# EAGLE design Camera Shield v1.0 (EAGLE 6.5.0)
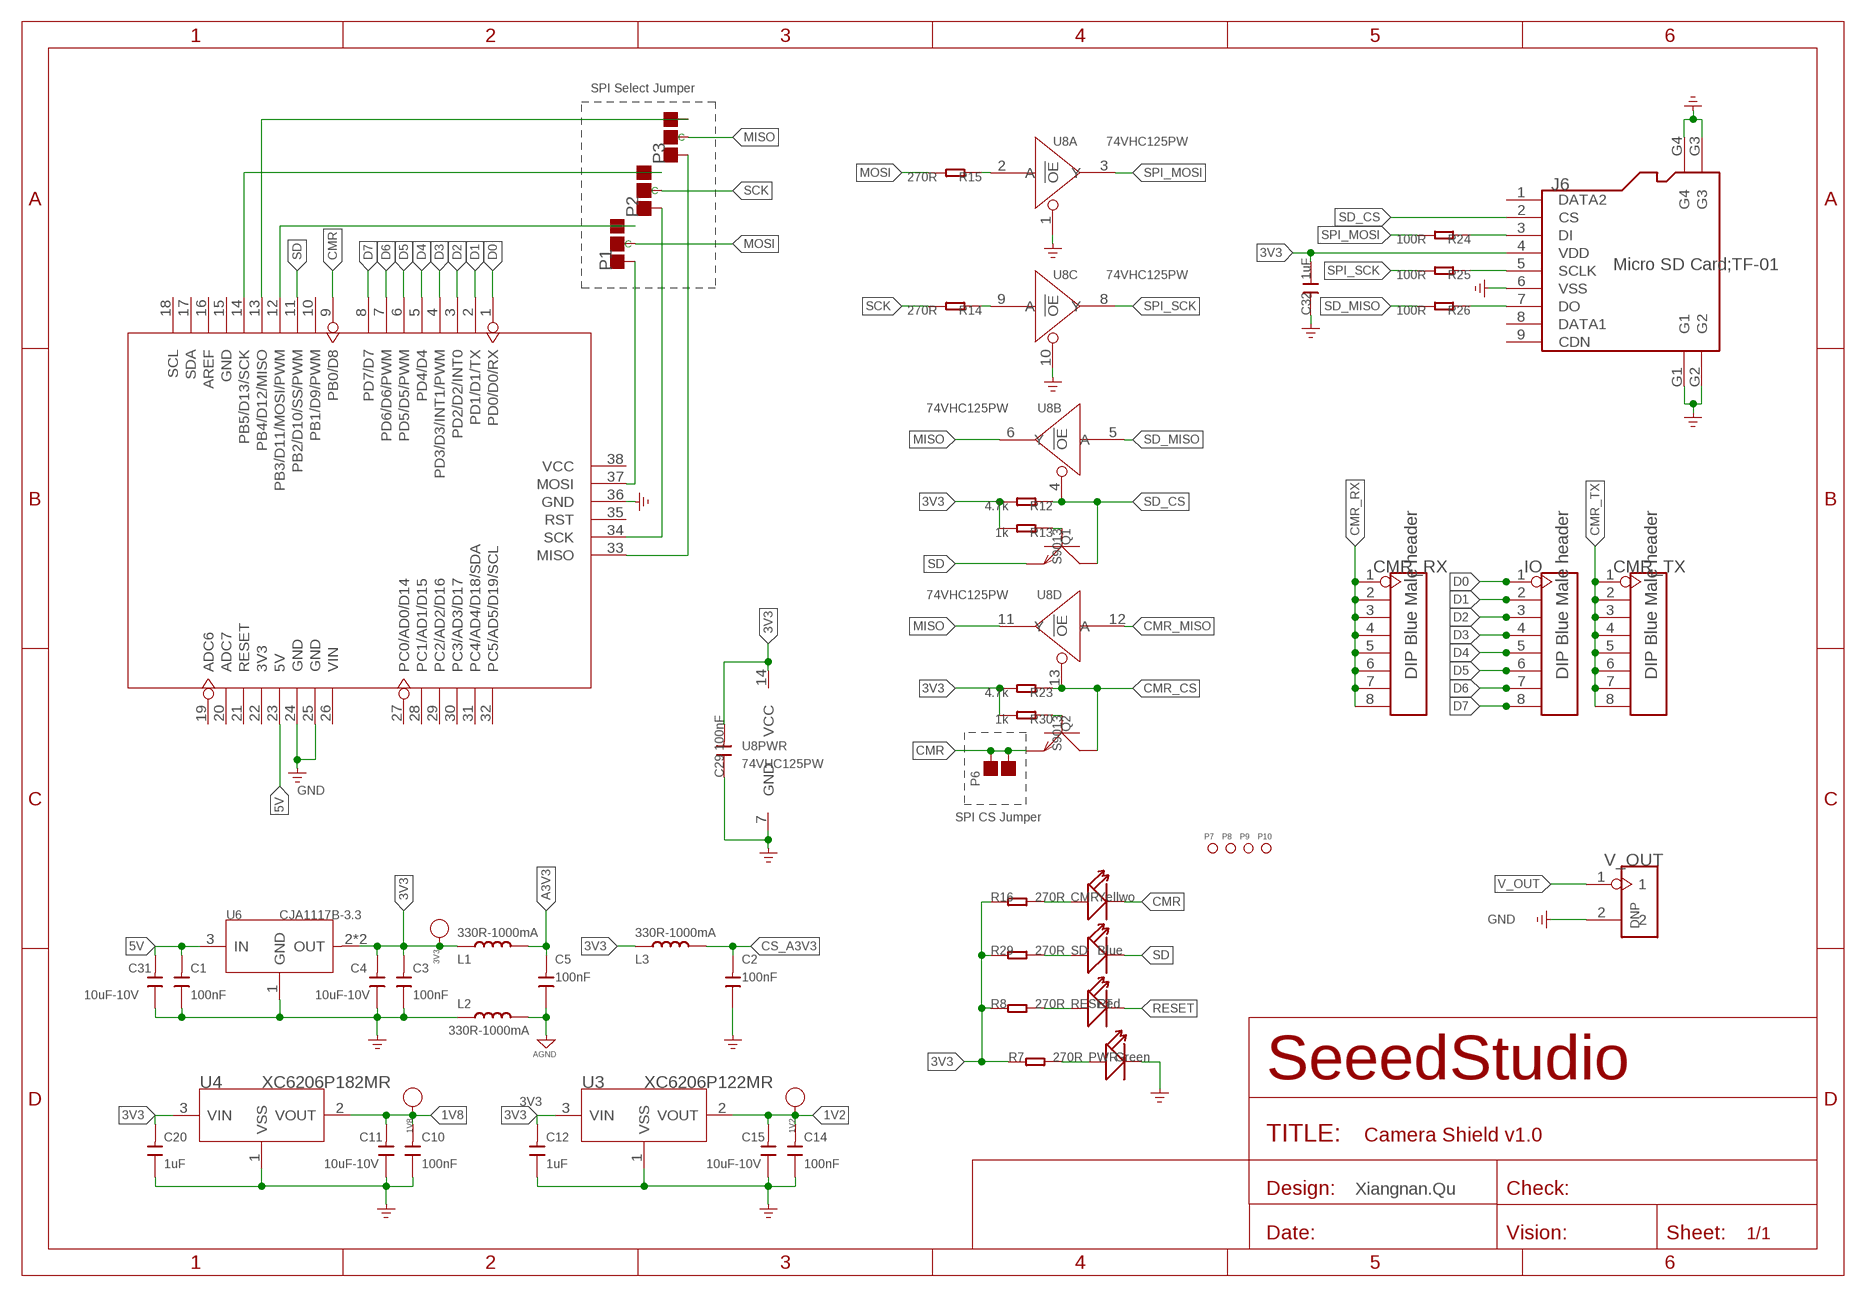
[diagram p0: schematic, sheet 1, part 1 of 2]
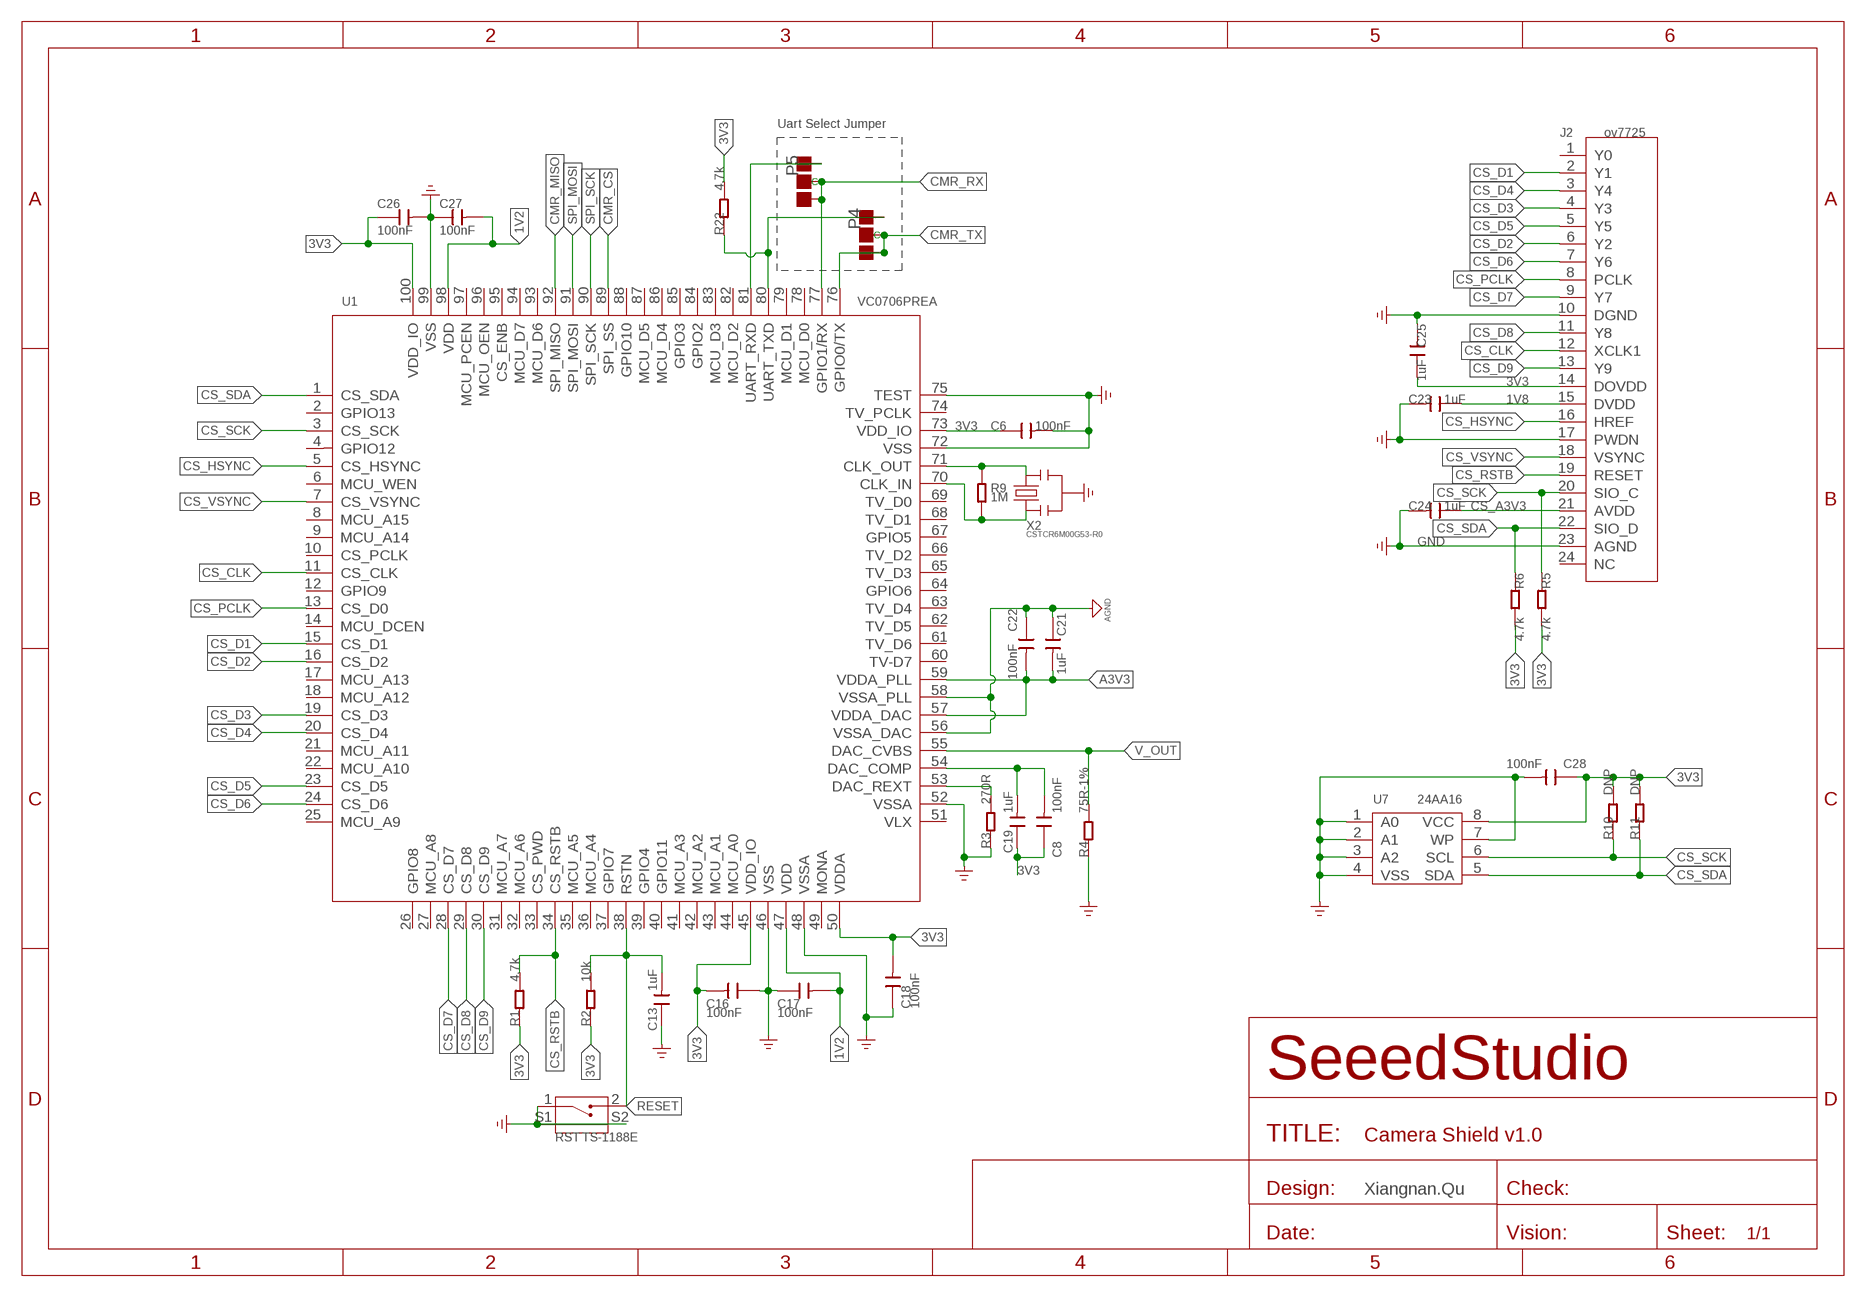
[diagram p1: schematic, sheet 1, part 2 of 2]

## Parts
1V2  PAD-TEST-POINT'4545'  [TP_4545]
1V8  PAD-TEST-POINT'4545'  [TP_4545]
3V3  PAD-TEST-POINT'4545'  [TP_4545]
C1  100nF  C-0603  [C0603]
C2  100nF  C-0603  [C0603]
C3  100nF  C-0603  [C0603]
C4  10uF-10V  C-0805  [C0805]
C5  100nF  C-0603  [C0603]
C6  100nF  C-0603  [C0603]
C8  100nF  C-0603  [C0603]
C10  100nF  C-0603  [C0603]
C11  10uF-10V  C-0805  [C0805]
C12  1uF  C-0603  [C0603]
C13  1uF  C-0603  [C0603]
C14  100nF  C-0603  [C0603]
C15  10uF-10V  C-0805  [C0805]
C16  100nF  C-0603  [C0603]
C17  100nF  C-0603  [C0603]
C18  100nF  C-0603  [C0603]
C19  1uF  C-0603  [C0603]
C20  1uF  C-0603  [C0603]
C21  1uF  C-0603  [C0603]
C22  100nF  C-0603  [C0603]
C23  1uF  C-0603  [C0603]
C24  1uF  C-0603  [C0603]
C25  1uF  C-0603  [C0603]
C26  100nF  C-0603  [C0603]
C27  100nF  C-0603  [C0603]
C28  100nF  C-0603  [C0603]
C29  100nF  C-0603  [C0603]
C31  10uF-10V  C-0805  [C0805]
C32  1uF  C-0603  [C0603]
CMR  Yellwo  LED'0603'  [LED-0603]
CMR_RX  DIP Blue Male header  HEADER-8P-2.54  [8P-2.54]
CMR_TX  DIP Blue Male header  HEADER-8P-2.54  [8P-2.54]
IO  DIP Blue Male header  HEADER-8P-2.54  [8P-2.54]
J2  ov7725  CAMERA-OV7670  [24P-0.5-16.2X5.8X2.0H]
J6  Micro SD Card;TF-01  HOLDER-MICROSD-9P'HOLDER'  [9P-SMD-W/-RING]
L1  330R-1000mA  L'0603'  [L0603]
L2  330R-1000mA  L'0603'  [L0603]
L3  330R-1000mA  L'0603'  [L0603]
P1  PAD-JUMPER-3P-40*40  [3P-SMD-4.1X1.5]
P2  PAD-JUMPER-3P-40*40  [3P-SMD-4.1X1.5]
P3  PAD-JUMPER-3P-40*40  [3P-SMD-4.1X1.5]
P4  PAD-JUMPER-3P-40*40  [3P-SMD-4.1X1.5]
P5  PAD-JUMPER-3P-40*40  [3P-SMD-4.1X1.5]
P6  PAD-JUMPER-2P  [2P-SMD-1.78X1.27]
P7  PAD-MARK'ANNULAR'  [ROUND-MARK-1.0]
P8  PAD-MARK'ANNULAR'  [ROUND-MARK-1.0]
P9  PAD-MARK'ANNULAR'  [ROUND-MARK-1.0]
P10  PAD-MARK'ANNULAR'  [ROUND-MARK-1.0]
PWR  Green  LED'0603'  [LED-0603]
Q1  S9013  TRANSISTOR-NPN-SOT23  [SOT23]
Q2  S9013  TRANSISTOR-NPN-SOT23  [SOT23]
R1  4.7k  R-0603  [R0603]
R2  10k  R-0603  [R0603]
R3  270R  R-0603  [R0603]
R4  75R-1%  R-0603  [R0603]
R5  4.7k  R-0603  [R0603]
R6  4.7k  R-0603  [R0603]
R7  270R  R-0603  [R0603]
R8  270R  R-0603  [R0603]
R9  1M  R-0603  [R0603]
R10  DNP  R-0603  [R0603]
R11  DNP  R-0603  [R0603]
R12  4.7k  R-0603  [R0603]
R13  1k  R-0603  [R0603]
R14  270R  R-0603  [R0603]
R15  270R  R-0603  [R0603]
R16  270R  R-0603  [R0603]
R22  4.7k  R-0603  [R0603]
R23  4.7k  R-0603  [R0603]
R24  100R  R-0603  [R0603]
R25  100R  R-0603  [R0603]
R26  100R  R-0603  [R0603]
R29  270R  R-0603  [R0603]
R30  1k  R-0603  [R0603]
RESET  Red  LED'0603'  [LED-0603]
RST  TS-1188E  BUTTON-2P-REINFORCE-3100060P1  [4P-SMD-7.0X3.5X3.5H-90D]
SD  Blue  LED'0603'  [LED-0603]
U1  VC0706PREA  VC0706'PREA'  [LQFP100]
U3  XC6206P122MR  XC6206MR  [SOT23]
U4  XC6206P182MR  XC6206MR  [SOT23]
U5  ARDUINO-38P'WITH/-SILK'  [ARDUINO-38P-WITH/-SILK-500519002]
U6  CJA1117B-3.3  LD1117'SOT89'  [SOT89]
U7  24AA16  CAT24C256  [SOIC8-6.0]
U8  74VHC125PW  [TSSOP14]
V_OUT  DNP  HEADER-2P-65/35MIL  [2P-2.54-65/35MIL]
X2  CSTCR6M00G53-R0  CRYSTAL-RESONATOR'CSTCR6M00G53-R0'  [3P-SMD-4.5X2.0X1.2H]

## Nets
1V2: 1V2.T C14.2 C15.2 C17.2 C27.2 U1.47(VDD) U1.98(VDD) U3.2(VOUT)
1V8: 1V8.T C10.2 C11.2 C23.1 J2.15(DVDD) U4.2(VOUT)
3V3: 3V3.T C3.2 C4.2 C6.1 C8.1 C12.2 C16.2 C18.2 C19.1 C20.2 C25.1 C26.1 C28.1 C29.2 C32.1 J2.14(DOVDD) J6.4(VDD) L1.1 L3.1 R1.1 R2.1 R5.2 R6.2 R7.1 R8.1 R10.2 R11.2 R12.2 R13.2 R16.1 R22.2 R23.2 R29.1 R30.2 U1.45(VDD_IO) U1.50(VDDA) U1.73(VDD_IO) U1.100(VDD_IO) U3.3(VIN) U4.3(VIN) U6.2(OUT) U6.4(OUT) U7.8(VCC) U8.14(PWR:VCC)
5V: C1.2 C31.2 U5.23(5V) U6.3(IN)
A3V3: C5.2 C21.2 C22.2 L1.2 U1.57(VDDA_DAC) U1.59(VDDA_PLL)
AGND: C5.1 C21.1 C22.1 L2.2 U1.56(VSSA_DAC) U1.58(VSSA_PLL)
CMR: CMR.- P6.1 P6.2 Q2.2(E) U5.9(PB0/D8)
CMR_CS: Q2.3(C) R23.1 U1.89(SPI_SS) U8.13(D:!OE)
CMR_MISO: U1.92(SPI_MISO) U8.12(D:A)
CMR_RX: CMR_RX.1 CMR_RX.2 CMR_RX.3 CMR_RX.4 CMR_RX.5 CMR_RX.6 CMR_RX.7 CMR_RX.8 P5.00(L) P5.MM(C) U1.77(GPIO1/RX)
CMR_TX: CMR_TX.1 CMR_TX.2 CMR_TX.3 CMR_TX.4 CMR_TX.5 CMR_TX.6 CMR_TX.7 CMR_TX.8 P4.00(L) P4.MM(C) U1.76(GPIO0/TX)
CS_A3V3: C2.2 C24.1 J2.21(AVDD) L3.2
CS_CLK: J2.12(XCLK1) U1.11(CS_CLK)
CS_D1: J2.2(Y1) U1.15(CS_D1)
CS_D2: J2.6(Y2) U1.16(CS_D2)
CS_D3: J2.4(Y3) U1.19(CS_D3)
CS_D4: J2.3(Y4) U1.20(CS_D4)
CS_D5: J2.5(Y5) U1.23(CS_D5)
CS_D6: J2.7(Y6) U1.24(CS_D6)
CS_D7: J2.9(Y7) U1.28(CS_D7)
CS_D8: J2.11(Y8) U1.29(CS_D8)
CS_D9: J2.13(Y9) U1.30(CS_D9)
CS_HSYNC: J2.16(HREF) U1.5(CS_HSYNC)
CS_PCLK: J2.8(PCLK) U1.13(CS_D0)
CS_RSTB: J2.19(RESET) R1.2 U1.34(CS_RSTB)
CS_SCK: J2.20(SIO_C) R5.1 R10.1 U1.3(CS_SCK) U7.6(SCL)
CS_SDA: J2.22(SIO_D) R6.1 R11.1 U1.1(CS_SDA) U7.5(SDA)
CS_VSYNC: J2.18(VSYNC) U1.7(CS_VSYNC)
D0: IO.1 U5.1(PD0/D0/RX)
D1: IO.2 U5.2(PD1/D1/TX)
D2: IO.3 U5.3(PD2/D2/INT0)
D3: IO.4 U5.4(PD3/D3/INT1/PWM)
D4: IO.5 U5.5(PD4/D4)
D5: IO.6 U5.6(PD5/D5/PWM)
D6: IO.7 U5.7(PD6/D6/PWM)
D7: IO.8 U5.8(PD7/D7)
D$2: J6.7(DO) R26.1
GND: C1.1 C2.1 C3.1 C4.1 C6.2 C10.1 C11.1 C12.1 C13.1 C14.1 C15.1 C16.1 C17.1 C18.1 C20.1 C23.2 C24.2 C25.2 C26.2 C27.1 C28.2 C29.1 C31.1 C32.2 J2.10(DGND) J2.17(PWDN) J2.23(AGND) J6.6(VSS) J6.G1 J6.G2 J6.G3 J6.G4 L2.1 PWR.- R3.1 R4.1 RST.1 RST.S1 RST.S2 U1.46(VSS) U1.48(VSSA) U1.52(VSSA) U1.72(VSS) U1.75(TEST) U1.99(VSS) U3.1(VSS) U4.1(VSS) U5.24(GND) U5.25(GND) U5.36(GND) U6.1(GND) U7.1(A0) U7.2(A1) U7.3(A2) U7.4(VSS) U7.7(WP) U8.1(A:!OE) U8.7(PWR:GND) U8.10(C:!OE) V_OUT.2 X2.2
MISO: P3.MM(C) U8.6(B:Y) U8.11(D:Y)
MISOP: P3.00(L) U5.13(PB4/D12/MISO)
MISOT: P3.11(R) U5.33(MISO)
MOSI: P1.MM(C) R15.2
MOSIP: P1.00(L) U5.12(PB3/D11/MOSI/PWM)
N$1: R3.2 U1.53(DAC_REXT)
N$2: R9.1 U1.70(CLK_IN) X2.1
N$3: P2.11(R) U5.34(SCK)
N$4: CMR.+ R16.2
N$5: P4.11(R) R22.1 U1.80(UART_TXD)
N$6: R15.1 U8.2(A:A)
N$7: R14.1 U8.9(C:A)
N$8: P1.11(R) U5.37(MOSI)
N$9: PWR.+ R7.2
N$10: R8.2 RESET.+
N$11: Q2.1(B) R30.1
N$12: J6.3(DI) R24.1
N$13: J6.5(SCLK) R25.1
N$14: R29.2 SD.+
N$18: Q1.1(B) R13.1
N$24: P5.11(R) U1.81(UART_RXD)
N$32: C8.2 C19.2 U1.54(DAC_COMP)
N$37: R9.2 U1.71(CLK_OUT) X2.3
RESET: C13.2 R2.2 RESET.- RST.2 U1.38(RSTN)
SCK: P2.MM(C) R14.2
SCKP: P2.00(L) U5.14(PB5/D13/SCK)
SD: Q1.2(E) SD.- U5.11(PB2/D10/SS/PWM)
SD_CS: J6.2(CS) Q1.3(C) R12.1 U8.4(B:!OE)
SD_MISO: R26.2 U8.5(B:A)
SPI_MOSI: R24.2 U1.91(SPI_MOSI) U8.3(A:Y)
SPI_SCK: R25.2 U1.90(SPI_SCK) U8.8(C:Y)
V_OUT: R4.2 U1.55(DAC_CVBS) V_OUT.1
Unconnected: J2.1(Y0) J2.24(NC) J6.1(DATA2) J6.8(DATA1) J6.9(CDN) U1.2(GPIO13) U1.4(GPIO12) U1.6(MCU_WEN) U1.8(MCU_A15) U1.9(MCU_A14) U1.10(CS_PCLK) U1.12(GPIO9) U1.14(MCU_DCEN) U1.17(MCU_A13) U1.18(MCU_A12) U1.21(MCU_A11) U1.22(MCU_A10) U1.25(MCU_A9) U1.26(GPIO8) U1.27(MCU_A8) U1.31(MCU_A7) U1.32(MCU_A6) U1.33(CS_PWD) U1.35(MCU_A5) U1.36(MCU_A4) U1.37(GPIO7) U1.39(GPIO4) U1.40(GPIO11) U1.41(MCU_A3) U1.42(MCU_A2) U1.43(MCU_A1) U1.44(MCU_A0) U1.49(MONA) U1.51(VLX) U1.60(TV-D7) U1.61(TV_D6) U1.62(TV_D5) U1.63(TV_D4) U1.64(GPIO6) U1.65(TV_D3) U1.66(TV_D2) U1.67(GPIO5) U1.68(TV_D1) U1.69(TV_D0) U1.74(TV_PCLK) U1.78(MCU_D0) U1.79(MCU_D1) U1.82(MCU_D2) U1.83(MCU_D3) U1.84(GPIO2) U1.85(GPIO3) U1.86(MCU_D4) U1.87(MCU_D5) U1.88(GPIO10) U1.93(MCU_D6) U1.94(MCU_D7) U1.95(CS_ENB) U1.96(MCU_OEN) U1.97(MCU_PCEN) U5.10(PB1/D9/PWM) U5.15(GND) U5.16(AREF) U5.17(SDA) U5.18(SCL) U5.19(ADC6) U5.20(ADC7) U5.21(RESET) U5.22(3V3) U5.26(VIN) U5.27(PC0/AD0/D14) U5.28(PC1/AD1/D15) U5.29(PC2/AD2/D16) U5.30(PC3/AD3/D17) U5.31(PC4/AD4/D18/SDA) U5.32(PC5/AD5/D19/SCL) U5.35(RST) U5.38(VCC)

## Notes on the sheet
- SPI Select Jumper
- Uart Select Jumper
- SPI CS Jumper
- Xiangnan.Qu | Xiangnan.Qu

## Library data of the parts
1V2 1V8 3V3 = Discrete:PAD-TEST-POINT; PARTNO: DNP
C1-C6 C8 C10-C29 C31 C32 = Discrete:C*: Ceramic Capacitors
CMR PWR RESET SD = Discrete:LED*
CMR_RX CMR_TX IO = Connector:HEADER-8P
J2 = template:CAMERA-OV7670
J6 = Connector:HOLDER-MICROSD-9P
L1-L3 = Discrete:L*
P1-P5 = Discrete:PAD-JUMPER-3P; PARTNO: DNP
P6 = Discrete:PAD-JUMPER-2P; PARTNO: DNP
P7-P10 = Discrete:PAD-MARK; PARTNO: DNP
Q1 Q2 = Discrete:TRANSISTOR-NPN*: NPN audion
R1-R16 R22-R26 R29 R30 = Discrete:R*
RST = Discrete:BUTTON-2P-REINFORCE: TS-1188E http://www.best-dz.com/?thread-374-2.html SMD Button
U1 = template:VC0706
U3 U4 = IC:XC6206: LOW ESR Cap.Compatible Positive Voltage Regulators
U5 = moudle:ARDUINO-38P
U6 = IC:LD1117: Low Drop Fixed And Adjustable Positive Voltage Regulators http://www.datasheetcatalog.org/datasheet/SGSThomsonMicroelectronics/mXuqtqv.pdf
U7 = IC:CAT24C256: 256 kb I2C CMOS Serial EEPROM
U8 = IC:74V*125: Quad Buffer/Line Driver;3-state
V_OUT = Connector:HEADER-2P
X2 = Discrete:CRYSTAL-RESONATOR: Resonator Small SMD resonator. This is the itty bitty 10/20MHz resonators with built in caps. CSTCE10M0G55 and CSTCE20M0V53. Footprint has been reviewed closely but hasn't been tested yet.

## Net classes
0 default: width 0.152 mm, drill 0.305 mm, clearance 0.152 mm

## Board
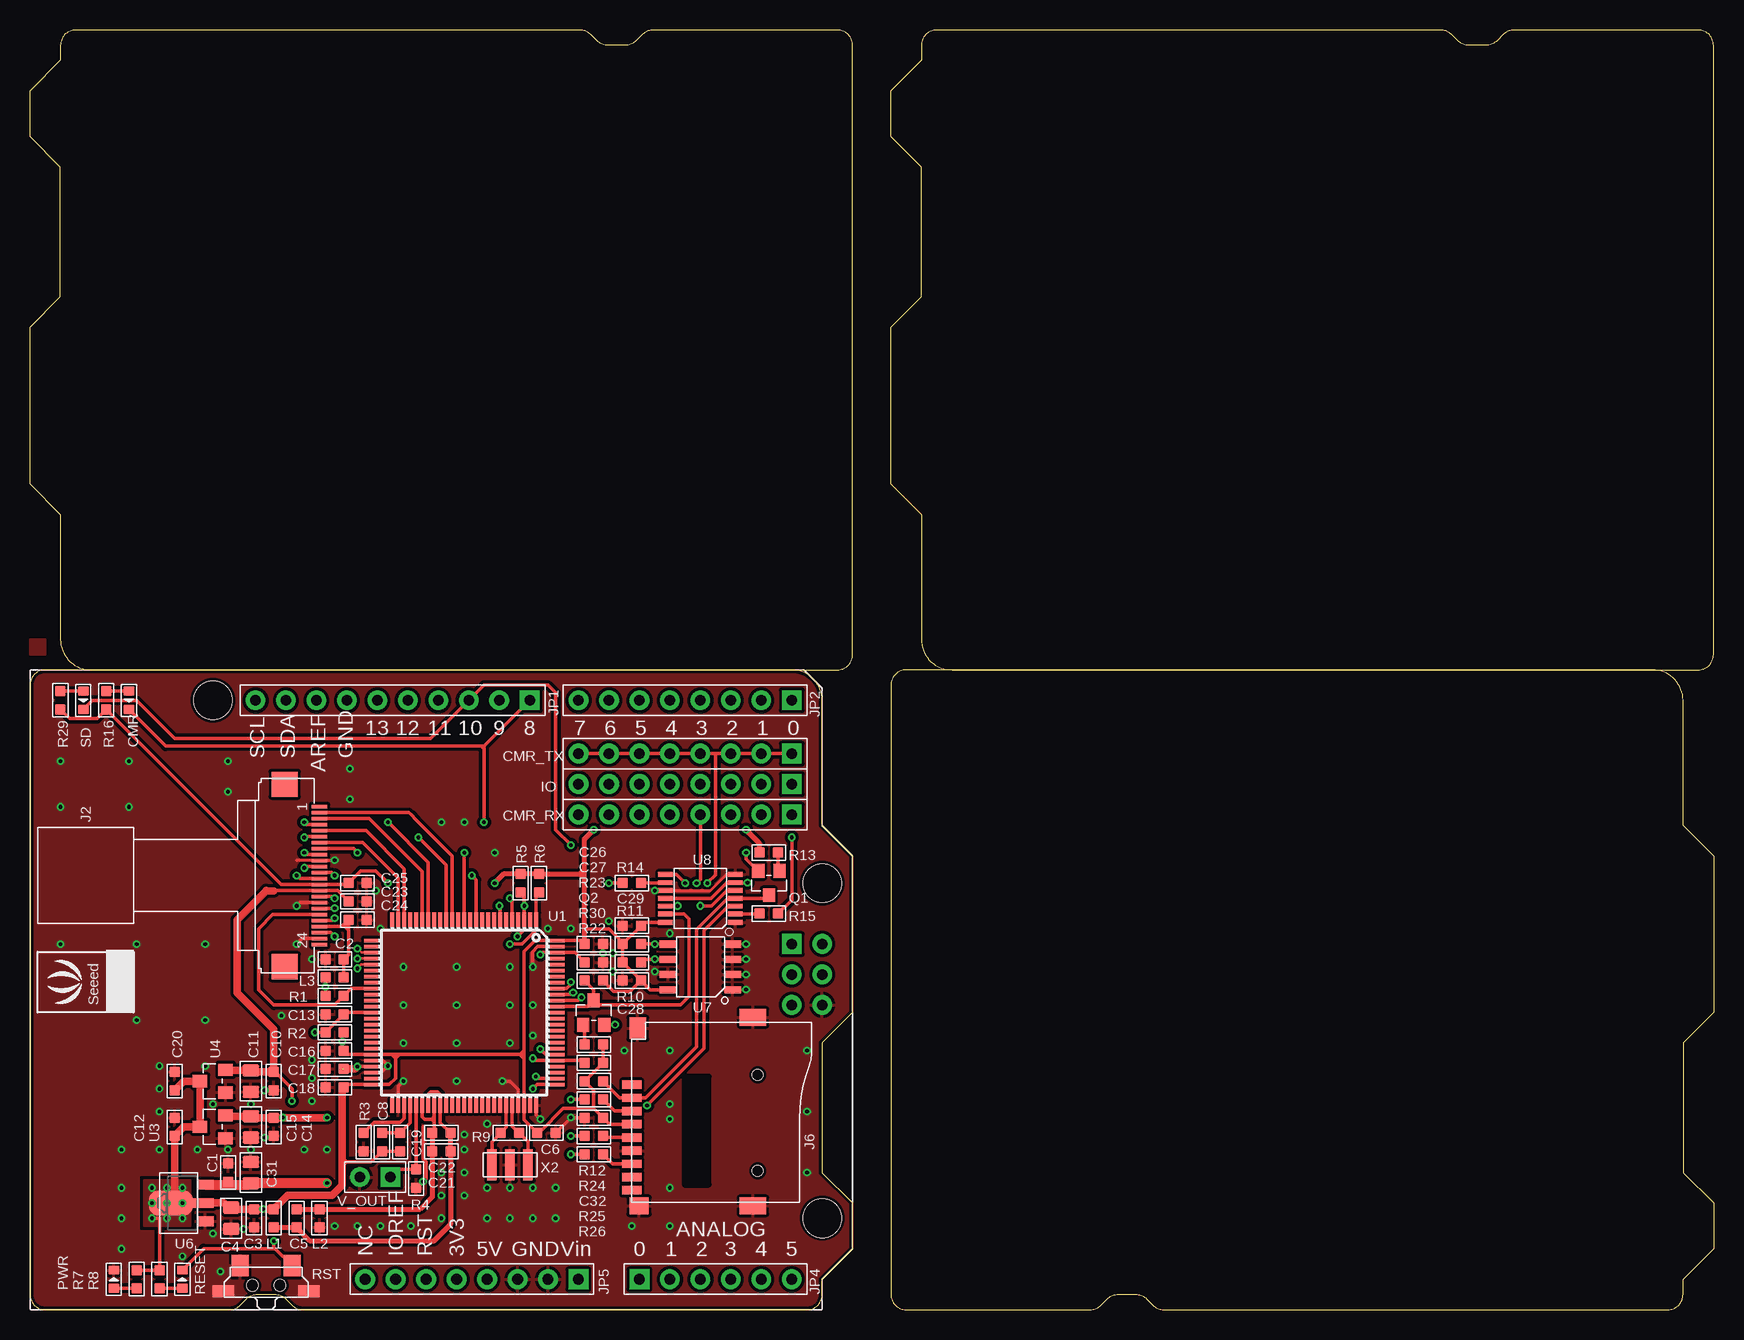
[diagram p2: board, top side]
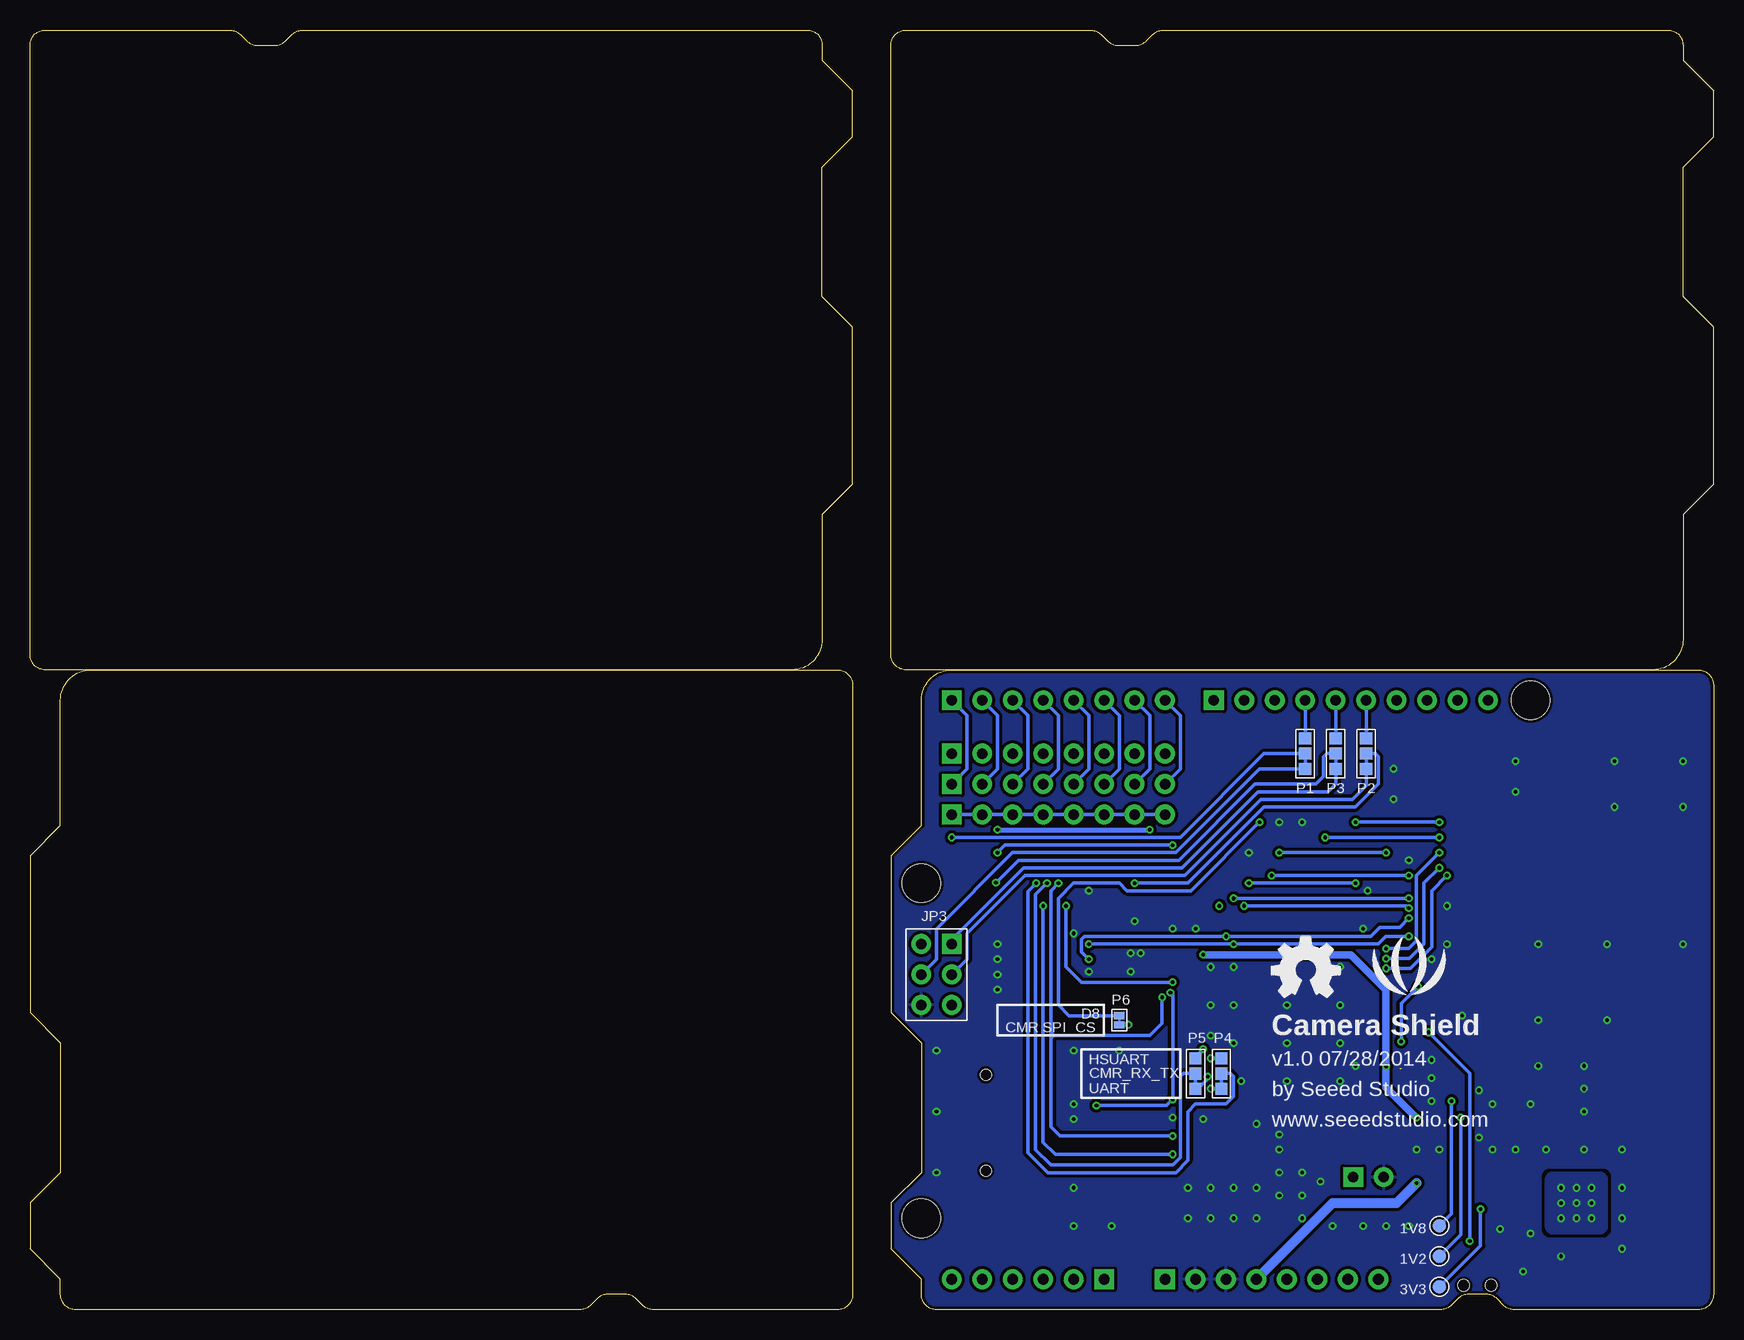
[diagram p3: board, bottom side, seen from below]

Size 140.34 x 106.68 mm. Coordinates in mm from the lower left corner, seen from the top.
Outline: 96 segments
Copper layers (1*16): Top 0.035mm / dielectric 1.5mm / Bottom 0.035mm
Design rules "SeeedStudio_2layer_DRU_no_angle_20140221 *": minimum track width 6mil, minimum drill 12mil, track to track 6mil, track to pad 6mil, pad to pad 6mil, via to via 6mil, smd to smd 0mil, copper to edge 10mil, drill to drill 10mil, minimum pad ring 10mil, minimum via ring 6mil, stop-mask expansion 2mil, vias tented up to drill 100mil, thermal gap 10mil
Holes 2.03 mm at 7.62,111.12 132.72,111.12 132.72,-4.45 7.62,-4.45

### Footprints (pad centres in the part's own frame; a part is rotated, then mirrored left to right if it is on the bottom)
TP_4545 = smd 1.143 x 1.143: T 0,0
C0603 = smd 0.889 x 0.889: 1 -0.762,0; 2 0.762,0
C0805 = smd 1.016 x 1.397: 1 -0.889,0; 2 0.889,0
LED-0603 = smd 0.762 x 0.889: + -0.762,0; - 0.762,0
8P-2.54 = drill 0.889 pad 1.651 square: 1 0,8.89 | drill 0.889 pad 1.651: 2 0,6.35; 3 0,3.81; 4 0,1.27; 5 0,-1.27; 6 0,-3.81; 7 0,-6.35; 8 0,-8.89
24P-0.5-16.2X5.8X2.0H = smd 0.3 x 1.3: 1 -5.75,0; 2 -5.25,0; 3 -4.75,0; 4 -4.25,0; 5 -3.75,0; 6 -3.25,0; 7 -2.75,0; 8 -2.25,0; 9 -1.75,0; 10 -1.25,0; 11 -0.75,0; 12 -0.25,0; 13 0.25,0; 14 0.75,0; 15 1.25,0; 16 1.75,0; 17 2.25,0; 18 2.75,0; 19 3.25,0; 20 3.75,0; 21 4.25,0; 22 4.75,0; 23 5.25,0; 24 5.75,0 | smd 2.1 x 2.2: P1 -7.6,-2.9; P2 7.6,-2.9
9P-SMD-W/-RING = smd 1.6 x 0.7: 1 0,2.25; 2 0,1.15; 3 0,0.05; 4 0,-1.05; 5 0,-2.15; 6 0,-3.25; 7 0,-4.35; 8 0,-5.45; 9 0,-6.55 | smd 1.6 x 1.4: G1 0.6,-7.85 | smd 2.2 x 1.4: G2 10.1,-7.85; G3 10.1,7.85 | smd 1.4 x 1.8: G4 0.5,6.95 | hole 0.9: 10.5,-4.95; 10.5,3.05
L0603 = smd 0.889 x 0.889: 1 -0.762,0; 2 0.762,0
3P-SMD-4.1X1.5 = smd 1.016 x 1.016: 00 -1.27,0; 11 1.27,0; MM 0,0
2P-SMD-1.78X1.27 = smd 0.889 x 0.61: 1 0,0.381; 2 0,-0.381
ROUND-MARK-1.0 = smd 1.016 x 1.016: P$1 0,0
SOT23 = smd 1.016 x 1.143: 1 -0.889,-1.016; 2 0.889,-1.016; 3 0,1.016
R0603 = smd 0.889 x 0.889: 1 -0.762,0; 2 0.762,0
4P-SMD-7.0X3.5X3.5H-90D = smd 1.397 x 1.778: 1 -2.159,1.651; 2 2.159,1.651 | smd 1.778 x 1.016: S1 -3.556,-0.508; S2 3.556,-0.508 | hole 0.95: -1.15,0; 1.15,0
LQFP100 = smd 1.2 x 0.32: 1 -7.75,6; 2 -7.75,5.5; 3 -7.75,5; 4 -7.75,4.5; 5 -7.75,4; 6 -7.75,3.5; 7 -7.75,3; 8 -7.75,2.5; 9 -7.75,2; 10 -7.75,1.5; 11 -7.75,1; 12 -7.75,0.5; 13 -7.75,0; 14 -7.75,-0.5; 15 -7.75,-1; 16 -7.75,-1.5; 17 -7.75,-2; 18 -7.75,-2.5; 19 -7.75,-3; 20 -7.75,-3.5; 21 -7.75,-4; 22 -7.75,-4.5; 23 -7.75,-5; 24 -7.75,-5.5; 25 -7.75,-6; 51 7.75,-6; 52 7.75,-5.5; 53 7.75,-5; 54 7.75,-4.5; 55 7.75,-4; 56 7.75,-3.5; 57 7.75,-3; 58 7.75,-2.5; 59 7.75,-2; 60 7.75,-1.5; 61 7.75,-1; 62 7.75,-0.5; 63 7.75,0; 64 7.75,0.5; 65 7.75,1; 66 7.75,1.5; 67 7.75,2; 68 7.75,2.5; 69 7.75,3; 70 7.75,3.5; 71 7.75,4; 72 7.75,4.5; 73 7.75,5; 74 7.75,5.5; 75 7.75,6 | smd 0.32 x 1.2: 26 -6,-7.75; 27 -5.5,-7.75; 28 -5,-7.75; 29 -4.5,-7.75; 30 -4,-7.75; 31 -3.5,-7.75; 32 -3,-7.75; 33 -2.5,-7.75; 34 -2,-7.75; 35 -1.5,-7.75; 36 -1,-7.75; 37 -0.5,-7.75; 38 0,-7.75; 39 0.5,-7.75; 40 1,-7.75; 41 1.5,-7.75; 42 2,-7.75; 43 2.5,-7.75; 44 3,-7.75; 45 3.5,-7.75; 46 4,-7.75; 47 4.5,-7.75; 48 5,-7.75; 49 5.5,-7.75; 50 6,-7.75; 76 6,7.75; 77 5.5,7.75; 78 5,7.75; 79 4.5,7.75; 80 4,7.75; 81 3.5,7.75; 82 3,7.75; 83 2.5,7.75; 84 2,7.75; 85 1.5,7.75; 86 1,7.75; 87 0.5,7.75; 88 0,7.75; 89 -0.5,7.75; 90 -1,7.75; 91 -1.5,7.75; 92 -2,7.75; 93 -2.5,7.75; 94 -3,7.75; 95 -3.5,7.75; 96 -4,7.75; 97 -4.5,7.75; 98 -5,7.75; 99 -5.5,7.75; 100 -6,7.75
SOT23' = smd 1.016 x 1.2: 1 -0.95,-1.06; 2 0.95,-1.06; 3 0,1.06
ARDUINO-38P-WITH/-SILK-500519002 = drill 0.889 pad 1.651 square: 1 63.5,50.8; 9 41.656,50.8; 26 45.72,2.54; 27 50.8,2.54; 33 63.5,30.48 | drill 0.889 pad 1.651: 2 60.96,50.8; 3 58.42,50.8; 4 55.88,50.8; 5 53.34,50.8; 6 50.8,50.8; 7 48.26,50.8; 8 45.72,50.8; 10 39.116,50.8; 11 36.576,50.8; 12 34.036,50.8; 13 31.496,50.8; 14 28.956,50.8; 15 26.416,50.8; 16 23.876,50.8; 17 21.336,50.8; 18 18.796,50.8; 19 27.94,2.54; 20 30.48,2.54; 21 33.02,2.54; 22 35.56,2.54; 23 38.1,2.54; 24 40.64,2.54; 25 43.18,2.54; 28 53.34,2.54; 29 55.88,2.54; 30 58.42,2.54; 31 60.96,2.54; 32 63.5,2.54; 34 63.5,27.94; 35 63.5,25.4; 36 66.04,25.4; 37 66.04,27.94; 38 66.04,30.48 | hole 3.2: 15.24,50.8; 66.04,35.56; 66.04,7.62
SOT89 = smd 0.8 x 1.4: 1 -1.524,-1.905; 3 1.524,-1.905 | smd 0.8 x 1.9: 2 0,-1.651 | smd 2.032 x 3.65: 4 0,0.94
SOIC8-6.0 = smd 0.6 x 1.4: 1 -1.905,-2.7; 2 -0.635,-2.7; 3 0.635,-2.7; 4 1.905,-2.7; 5 1.905,2.7; 6 0.635,2.7; 7 -0.635,2.7; 8 -1.905,2.7
TSSOP14 = smd 0.4 x 1.2: 1 -2,-2.925; 2 -1.3,-2.925; 3 -0.65,-2.925; 4 0,-2.925; 5 0.65,-2.925; 6 1.3,-2.925; 7 2,-2.925; 8 2,2.925; 9 1.3,2.925; 10 0.65,2.925; 11 0,2.925; 12 -0.65,2.925; 13 -1.3,2.925; 14 -2,2.925
2P-2.54-65/35MIL = drill 0.889 pad 1.651 square: 1 0,1.27 | drill 0.889 pad 1.651: 2 0,-1.27
3P-SMD-4.5X2.0X1.2H = smd 0.8 x 2.6: 1 -1.5,0; 2 0,0; 3 1.5,0

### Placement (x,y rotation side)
1V2  22.86,4.45 0 bottom
1V8  22.86,6.99 0 bottom
3V3  22.86,1.91 0 bottom
C1  16.51,11.43 270 top
C2  25.4,29.21 0 top
C3  18.67,7.62 90 top
C4  16.76,7.62 90 top
C5  22.23,7.62 270 top
C6  43.05,14.73 0 top
C8  29.34,13.97 90 top
C10  20.32,19.05 90 top
C11  18.41,19.05 90 top
C12  12.06,15.24 270 top
C13  25.4,24.64 0 top
C14  20.32,15.24 90 top
C15  18.41,15.24 90 top
C16  25.4,21.59 0 top
C17  25.4,20.07 0 top
C18  25.4,18.54 0 top
C19  30.86,13.97 90 top
C20  12.06,19.05 270 top
C21  34.29,13.21 0 top
C22  34.29,14.73 0 top
C23  27.3,34.04 0 top
C24  27.3,32.51 0 top
C25  27.3,35.56 0 top
C26  46.99,30.48 0 top
C27  46.99,28.96 180 top
C28  50.16,27.43 180 top
C29  50.16,32 0 top
C31  18.41,11.43 270 top
C32  46.99,16 180 top
CMR  8.26,50.8 270 top
CMR_RX  54.61,41.27 270 top
CMR_TX  54.61,46.35 270 top
IO  54.61,43.81 270 top
J2  24.13,36.2 270 top
J6  50.16,16.51 0 top
L1  20.32,7.62 270 top
L2  24.13,7.62 90 top
L3  25.4,27.69 0 top
P1  34.04,46.35 270 bottom
P2  28.96,46.35 270 bottom
P3  31.5,46.35 270 bottom
P4  41.02,19.68 90 bottom
P5  43.18,19.68 90 bottom
P6  49.53,24.13 180 bottom
P7  not placed on the board
P8  not placed on the board
P9  not placed on the board
P10  not placed on the board
PWR  6.99,2.54 90 top
Q1  61.59,35.56 180 top
Q2  46.99,24.77 0 top
R1  25.4,26.16 0 top
R2  25.4,23.11 180 top
R3  27.81,13.97 90 top
R4  32.19,10.92 90 top
R5  40.89,35.56 90 top
R6  42.42,35.56 90 top
R7  8.89,2.54 270 top
R8  10.79,2.54 270 top
R9  40.01,14.73 0 top
R10  50.16,28.96 180 top
R11  50.16,30.48 180 top
R12  46.99,19.05 180 top
R13  61.59,38.1 180 top
R14  50.16,35.56 180 top
R15  61.59,33.02 0 top
R16  6.35,50.8 90 top
R22  46.99,20.57 0 top
R23  46.99,27.43 0 top
R24  46.99,17.53 180 top
R25  46.99,14.48 180 top
R26  46.99,12.95 180 top
R29  2.54,50.8 90 top
R30  46.99,22.1 0 top
RESET  12.7,2.54 90 top
RST  19.68,2.03 0 top
SD  4.45,50.8 270 top
U1  36.2,24.77 270 top
U3  XC6206P122MR  [SOT23']  15.24,15.24 90 top
U4  XC6206P182MR  [SOT23']  15.24,19.05 90 top
U5  0,0 0 top
U6  12.7,8.89 90 top
U7  55.88,28.57 90 top
U8  55.88,34.29 90 top
U$2  [SILK_SCREEN_150X124]  3.17,27.3 90 top
U$47  [LOGO_SILK]  25.4,27.94 0 bottom
U$52  [OSHW_FILLX200_NOTEXT]  36.83,26.04 0 bottom
V_OUT  28.77,11.05 270 top
X2  40.01,12.06 0 top

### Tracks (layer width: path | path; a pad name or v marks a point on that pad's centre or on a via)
1V2  (via drill 0.3 pad 0.64)  (1 unrouted)
  Top 0.305: U1.47 v27.3,20.27 | 26.36,20.27 C17.2 | v42.55,29.59 42.72,29.77 U1.98 45.42,29.77 C27.2
  Top 0.406: 20.19,16.13 C14.2 | 16.36,16.13 U3.2
  Top 0.61: 16.36,16.13 C15.2 18.54,16 C14.2 v21.08,16 v24.77,16 | v27.3,20.27 27.1,20.07 26.04,20.07
  Bottom 0.305: v27.3,20.27 | 1V2.T 21.08,6.22 v21.08,16
  Bottom 0.61: v24.77,16 27.3,18.54 v27.3,20.27 27.3,26.67 30.23,29.59 v42.55,29.59
1V8  (via drill 0.3 pad 0.64)
  Top 0.305: C23.1 25.63,34.95 J2.15 19.7,34.95 | C10.2 20.32,19.94 21.84,18.41 v21.84,17.4 | 18.54,19.81 C11.2 | 16.36,19.94 U4.2
  Top 0.61: 16.36,19.94 C11.2 | 18.54,19.81 C10.2 | 20.32,19.94 20.32,23.37 17.27,26.42 17.27,32.51 19.68,34.92 | 19.68,34.92 19.7,34.95 | 19.68,34.92 20.32,34.92
  Bottom 0.305: 1V8.T 21.84,8 v21.84,17.4
3V3  (via drill 0.3 pad 0.64)
  Top 0.305: R7.1 R8.1 10.79,7.62 v10.16,7.62 | C18.2 26.39,18.77 U1.50 29.94,18.77 30.48,19.3 30.48,20.95 | C19.1 C8.1 28.45,12.32 26.42,12.32 | 51.09,32.16 C29.2 | C28.1 R10.2 R11.2 | R11.2 C29.2 | 41.2,21.21 U1.73 41.2,15.83 C6.1 42.42,14.86 42.55,14.86 44.45,16.76 46.99,16.76 | 41.2,21.21 41.2,29.88 42.08,30.77 U1.100 46.07,30.77 46.23,30.61 | v29.84,35.56 28.83,36.58 27.56,36.58 C25.1 26.43,35.45 J2.14 20.94,35.45 R16.1 | R1.1 v24.64,26.92 L3.1 | U8.14 51.21,32.29 C29.2 | 30.17,21.27 U1.45 26.49,21.27 C16.2 26.04,21.46 v26.04,22.35 26.04,22.99 R2.1 | 30.17,21.27 30.48,21.27 | 30.48,21.27 40.85,21.27 | 40.85,21.27 41.14,21.27 41.2,21.21 | 30.48,20.95 30.48,21.27 | 30.23,21.21 30.48,20.95 | 30.48,20.95 30.73,21.21 30.23,21.21 | 30.17,21.27 30.23,21.21 | 40.85,21.27 40.85,21.29 41.15,21.59 41.15,20.95 40.85,21.26 40.85,21.27 | U7.8 51.69,26.67 C28.1 | 26.42,12.32 26.04,12.32 | 26.42,12.32 26.16,12.57 | 26.42,12.32 26.04,11.94 | J6.4 48.29,15.46 C32.1 47.62,16.13 | R30.2 R22.2 R12.2 46.99,18.29 46.99,16.76 | 47.62,16.13 46.99,16.76 | R16.1 6.35,50.16 | 2.41,49.91 R29.1 3.3,49.28 5.59,49.28 R16.1 | 47.62,16.13 47.62,15.88 | R11.2 49.4,30.61 48.26,31.75 46.48,31.75 | 46.48,31.75 46.23,31.75 | R23.2 47.88,27.43 47.88,27.3 48.64,26.54 50.04,26.54 C28.1 | 46.48,31.75 46.23,32 46.23,31.5 46.48,31.75
  Top 0.406: C18.2 26.04,18.54 | C26.1 46.23,30.61 46.23,31.5 46.23,31.75 46.23,32 46.23,35.94 | 46.23,35.94 46.23,36.45 | 46.23,36.45 46.23,36.7 | 46.23,36.7 46.23,39.24 v46.99,40.01 | v38.73,35.56 39.5,36.32 R5.2 R6.2 45.85,36.32 | R13.2 60.83,38.86 v59.69,40.01 | 45.85,36.32 46.1,36.32 46.23,36.45 | 45.85,36.32 46.23,36.7 | 45.85,36.32 46.23,35.94
  Top 0.61: C20.2 12.83,19.05 U4.3 U3.3 12.83,15.24 C12.2 12.06,9.2 U6.4 U6.2 16.13,8.89 16.51,8.51 C4.2 16.89,8.38 C3.2 v19.43,8.38 L1.1 21.46,9.53 25.18,9.53 26.04,10.38 26.04,11.94 26.04,12.32 26.04,18.54
  Bottom 0.305: v29.84,35.56 v38.73,35.56 | v26.04,22.35 26.04,25.53 v24.64,26.92 | 3V3.T 19.43,5.33 v19.43,8.38
  Bottom 0.406: v59.69,40.01 v46.99,40.01
  other vias: 10.16,10.16 11.43,10.16 12.7,10.16 12.7,8.89 10.16,8.89 11.43,7.62 11.43,8.89 12.7,7.62
  pour Bottom (isolate 0.254): 13.34,6.35 9.53,6.35 arc-90 8.89,6.99 8.89,10.79 arc-90 9.53,11.43 13.34,11.43 arc-90 13.97,10.79 13.97,6.99 arc-90
  pour Top (isolate 0.254, no thermals): 9.53,10.79 13.34,10.79 13.34,6.99 9.53,6.99
5V  (via drill 0.3 pad 0.64)
  Top 0.813: U6.3 16.51,10.41 | 16.51,10.41 18.29,10.41 C31.2 v24.77,10.54 | C1.2 16.51,10.41
  Bottom 0.813: U5.23 31.75,8.89 26.42,8.89 v24.77,10.54
A3V3
  Top 0.305: C22.2 34.2,15.59 U1.59 34.2,17.96 33.99,18.16 33.4,18.16 33.2,17.95 U1.57
  Top 0.406: L1.2 C5.2 23.37,5.71 33.66,5.71 35.05,7.11 C21.2 C22.2
AGND
  Top 0.305: U1.58 33.7,16.11 | 33.7,16.11 33.7,15.88 | 33.7,15.88 33.7,14.9 C22.1 | U1.56 32.7,16.07 32.89,15.88 33.47,15.88 | 33.47,15.88 33.7,15.88 | 33.7,16.11 33.47,15.88 | 33.47,15.88 33.66,15.68
  Top 0.406: C22.1 C21.1 33.53,9.4 32.51,8.38 L2.2 C5.1
CMR  (via drill 0.3 pad 0.64)
  Top 0.305: U5.9 37.85,46.99 | 37.85,46.99 37.59,46.99 | CMR.- 11.3,46.99 37.47,46.99 37.59,46.99 | v37.85,40.64 37.85,46.74 | 37.85,46.74 37.85,46.99 | 37.59,46.99 37.85,46.74 | v48.77,23.75 Q2.2
  Bottom 0.203: P6.1 P6.2
  Bottom 0.305: P6.2 53.72,24.51 54.61,25.4 54.61,34.29 53.34,35.56 49.53,35.56 48.9,34.92 43.56,34.92 v37.85,40.64 | P6.1 v48.77,23.75
CMR_CS
  Top 0.305: U1.89 46.47,25.27 46.86,25.65 | 46.86,25.65 Q2.3 46.99,26.67 R23.1 | U8.13 54.51,32.99 54.93,32.58 54.93,26.11 54.22,25.4 47.12,25.4 46.86,25.65
CMR_MISO  (via drill 0.3 pad 0.64)
  Top 0.305: U1.92 44.74,26.77 45.09,27.11 v45.09,27.3 | U8.12 53.96,33.64 v53.98,33.66
  Bottom 0.305: v53.98,33.66 53.98,28.57 52.7,27.3 v45.09,27.3
CMR_RX  (via drill 0.3 pad 0.64)
  Top 0.305: CMR_RX.4 55.88,35.88 v55.56,35.56 | U1.77 42.33,19.27 v42.16,19.43
  Bottom 0.305: CMR_RX.8 CMR_RX.7 CMR_RX.6 CMR_RX.5 CMR_RX.4 CMR_RX.3 CMR_RX.2 CMR_RX.1 | v55.56,35.56 56.52,34.61 56.52,13.34 55.24,12.06 45.09,12.06 44.45,12.7 44.45,19.43 44.2,19.68 P5.MM P5.00 42.99,18.41 42.16,19.24 v42.16,19.43
CMR_TX  (via drill 0.3 pad 0.64)
  Top 0.305: CMR_TX.8 CMR_TX.7 CMR_TX.6 CMR_TX.5 CMR_TX.4 57.15,46.35 | 57.15,46.35 CMR_TX.3 CMR_TX.2 CMR_TX.1 | 57.15,46.35 57.15,36.26 v56.45,35.56 | U1.76 42.26,18.77 v41.91,18.41
  Bottom 0.305: v56.45,35.56 57.15,34.86 57.15,13.08 55.5,11.43 44.83,11.43 43.81,12.45 43.81,16.51 43.18,17.14 40.64,17.14 40.01,17.78 40.01,19.43 40.26,19.68 P4.MM P4.00 v41.91,18.41
CS_A3V3
  Top 0.305: L3.2 C2.2 26.54,29.59 26.54,31.62 | C24.1 26.54,31.88 | J2.21 25.98,31.95 | 26.22,31.95 26.48,31.95 26.54,31.88 | 25.98,31.95 26.42,32.38 | 25.98,31.95 26.22,31.95 | 26.22,31.95 26.54,31.62 | 26.54,31.62 26.54,31.88
CS_CLK  (via drill 0.3 pad 0.64)
  Top 0.305: U1.11 37.2,35.83 v36.83,36.2 | J2.12 25.15,36.45 v25.4,36.2
  Bottom 0.305: v36.83,36.2 v25.4,36.2
CS_D1
  Top 0.305: U1.15 35.2,37.83 32.19,40.83 31.75,41.27 31.58,41.45 J2.2
CS_D2  (via drill 0.3 pad 0.64)
  Top 0.305: J2.6 22.93,39.45 v22.86,39.37 | v32.38,39.37 34.7,37.06 U1.16
  Bottom 0.305: v22.86,39.37 v32.38,39.37
CS_D3  (via drill 0.3 pad 0.64)
  Top 0.305: J2.4 23.05,40.45 v22.86,40.64 | v29.84,40.64 33.2,37.29 U1.19
  Bottom 0.305: v29.84,40.64 v22.86,40.64
CS_D4
  Top 0.305: U1.20 32.7,36.52 28.27,40.95 J2.3
CS_D5
  Top 0.305: U1.23 31.2,36.75 28,39.95 J2.5
CS_D6
  Top 0.305: U1.24 30.7,35.98 28.07,38.61 27.94,38.73 27.73,38.95 J2.7
CS_D7  (via drill 0.3 pad 0.64)
  Top 0.203: U1.28 27.64,29.77 v27.3,30.1
  Top 0.305: 22.99,37.97 v22.86,38.1 23.02,37.95 J2.9
  Bottom 0.305: v27.3,30.1 25.4,30.1 24.77,30.73 24.77,36.2 v22.86,38.1
CS_D8  (via drill 0.3 pad 0.64)
  Top 0.203: U1.29 27.31,29.27 v27.3,29.27
  Top 0.305: J2.11 22.98,36.95 v22.86,36.83
  Bottom 0.305: v27.3,29.27 25.34,29.27 24.13,30.48 24.13,35.56 v22.86,36.83
CS_D9  (via drill 0.3 pad 0.64)
  Top 0.203: U1.30 27.62,28.77 v27.3,28.45
  Top 0.305: J2.13 22.48,35.95 v22.23,36.2
  Bottom 0.305: v27.3,28.45 25.27,28.45 23.5,30.23 23.5,34.92 v22.23,36.2
CS_HSYNC  (via drill 0.3 pad 0.64)
  Top 0.305: J2.16 25.25,34.45 v25.4,34.29 | 40.13,34.16 v40.01,34.29 40.2,34.1 U1.5
  Bottom 0.305: v25.4,34.29 v40.01,34.29
CS_PCLK  (via drill 0.3 pad 0.64)
  Top 0.305: U1.13 v36.2,38.1 | 27.18,38.23 v27.3,38.1 26.96,38.45 J2.8
  Bottom 0.305: v36.2,38.1 v27.3,38.1
CS_RSTB
  Top 0.305: U1.34 26.77,26.77 R1.2 25.4,25.4 20.32,25.4 19.05,26.67 19.05,31.75 20.25,32.95 J2.19
CS_SCK  (via drill 0.3 pad 0.64)
  Top 0.305: R5.1 41.2,34.5 v41.2,33.66 U1.3 41.2,31.67 v40.64,31.11 | J2.20 25.21,32.45 v25.4,32.64 | U7.6 v52.07,29.21 51.18,29.21 R10.1
  Bottom 0.305: v25.4,32.64 26.16,31.88 27.81,31.88 28.57,31.11 40.26,31.11 v40.64,31.11 52.45,31.11 52.7,30.86 52.7,29.84 v52.07,29.21
CS_SDA  (via drill 0.3 pad 0.64)
  Top 0.305: R6.1 42.2,34.58 U1.1 42.2,31.65 41.02,30.48 v40.01,30.48 | U7.5 v52.07,30.48 R11.1 51.05,30.35 | J2.22 25.07,31.45 v25.4,31.11
  Bottom 0.305: v52.07,30.48 v40.01,30.48 27.94,30.48 27.3,31.11 v25.4,31.11
CS_VSYNC  (via drill 0.3 pad 0.64)
  Top 0.305: J2.18 25.38,33.45 v25.4,33.47 | U1.7 39.2,33.58 v39.12,33.66
  Bottom 0.305: v39.12,33.66 25.59,33.66 v25.4,33.47
D0
  Bottom 0.305: U5.1 62.23,49.53 62.23,45.09 IO.1
D1
  Bottom 0.305: IO.2 59.69,45.09 59.69,49.53 U5.2
D2
  Bottom 0.305: IO.3 57.15,45.09 57.15,49.53 U5.3
D3
  Bottom 0.305: IO.4 54.61,45.09 54.61,49.53 U5.4
D4
  Bottom 0.305: IO.5 52.07,45.09 52.07,49.53 U5.5
D5
  Bottom 0.305: IO.6 49.53,45.09 49.53,49.53 U5.6
D6
  Bottom 0.305: IO.7 46.99,45.09 46.99,49.53 U5.7
D7
  Bottom 0.305: IO.8 44.45,45.09 44.45,49.53 U5.8
D$2
  Top 0.305: J6.7 48.55,12.16 R26.1
GND  (via drill 0.3 pad 0.64)
  Top 0.254: J2.10 22.25,37.45 22.23,37.47 | U8.10 56.72,34.94 58.07,36.29 U8.7
  Top 0.305: J2.17 22.52,33.95 v22.23,33.66 | J2.10 25.38,37.45 v25.4,37.47 | J2.23 22.69,30.95 v22.23,30.48 | U1.46 29.4,20.77 v29.84,20.32 29.29,19.77 U1.48 | U1.52 30.7,18.63 v31.11,19.05 | U1.75 42.2,16.23 v42.55,15.88 | R4.1 32.26,10.16 33.02,10.92 33.02,12.32 32.77,12.57 32.77,15.24 | U1.99 42.33,30.27 41.91,29.84 v41.91,28.57 | U1.72 40.7,18.36 40.01,19.05 v39.37,19.05 | C32.2 v45.09,16 C6.2
  other vias: 29.21,31.75 28.83,34.92 35.56,19.05 25.4,6.99 38.1,15.49 36.2,14.61 36.2,13.34 36.2,11.43 43.81,10.16 38.1,10.16 41.91,10.16 38.1,7.62 29.21,6.99 31.75,6.99 34.29,11.43 34.29,9.53 34.29,7.62 52.07,34.92 23.5,17.4 23.5,19.3 19.56,18.29 18.41,17.14 18.41,13.34 16.51,13.34 10.79,16.51 14.61,20.32 15.24,17.14 23.5,29.21 48.26,32.38 10.79,13.34 10.79,18.41 10.79,20.32 7.62,13.34 7.62,10.16 7.62,7.62 15.24,6.35 7.62,5.08 31.11,22.23 35.56,22.23 31.11,28.57 35.56,28.57 40.01,28.57 35.56,25.4 31.11,25.4 38.73,38.1 41.91,7.62 43.81,7.62 50.16,6.99 64.77,21.59 64.77,16.51 64.77,11.43 14.61,30.48 16.51,43.18 16.51,45.72 14.61,24.13 24.77,13.34 22.86,13.34 47.75,29.72 49.53,21.59 53.34,15.88 53.34,17.14 59.69,30.48 59.69,29.21 59.69,27.94 59.69,26.67 45.09,31.75 43.18,31.75 53.34,21.59 36.2,9.53 40.01,7.62 40.01,10.16 15.88,3.17 17.78,6.73 12.7,4.45 27.3,6.99 32.77,10.67 53.34,10.16 53.34,6.99 41.91,25.4 41.91,22.86 40.01,22.23 40.01,25.4 48.58,28.19 48.58,29.72 52.07,28.19 13.97,13.34 53.34,31.37 36.2,40.64 34.29,40.64 26.67,45.09 26.67,42.55 2.54,45.72 8.26,45.72 8.26,41.91 2.54,41.91 8.89,30.48 2.54,30.48 8.89,24.13 23.5,20.83 19.56,14.35 20.95,24.51
  pour Top: 0,55.88 1.27,55.88 1.27,54.61 0,54.61
  pour Top (isolate 0.254, rank 2): 0,53.34 68.58,53.34 68.58,0 0,0
  pour Bottom (isolate 0.254, rank 2): 0,53.34 68.58,53.34 68.58,0 0,0
MISO  (via drill 0.3 pad 0.64)
  Top 0.305: U8.11 56.77,34.29 58.07,35.59 U8.6 v59.82,35.59
  Bottom 0.305: v59.82,35.59 57.94,37.47 44.58,37.47 38.23,43.81 33.15,43.81 32.51,44.45 32.51,46.07 32.23,46.35 P3.MM
MISOP
  Bottom 0.305: P3.00 U5.13
MISOT
  Bottom 0.305: U5.33 63.5,30.86 57.53,36.83 44.32,36.83 37.97,43.18 32.13,43.18 31.5,43.81 P3.11 31.5,46.35
MOSI  (via drill 0.3 pad 0.64)
  Top 0.305: v63.5,39.37 63.5,34.16 R15.2
  Bottom 0.305: v63.5,39.37 44.45,39.37 37.47,46.35 P1.MM
MOSIP
  Bottom 0.305: P1.00 U5.12
N$1
  Top 0.305: U1.53 31.2,15.96 30.86,15.62 28.7,15.62 R3.2
N$2
  Top 0.305: U1.70 39.7,15.18 R9.1 39.05,14.54 38.8,14.29 38.51,13.99 X2.1
N$3
  Bottom 0.305: U5.34 62.23,29.21 62.23,31.37 57.4,36.2 44.07,36.2 37.72,42.55 30.1,42.55 28.96,43.69 P2.11 28.96,46.35
N$4
  Top 0.305: CMR.+ R16.2
N$5  (via drill 0.3 pad 0.64)
  Top 0.305: R22.1 46.04,20.77 U1.80 42.1,20.77 v41.91,20.95
  Bottom 0.305: v41.91,20.95 P4.11
N$6
  Top 0.305: U8.2 60.8,32.99 R15.1
N$7
  Top 0.305: U8.9 50.96,35.59 R14.1
N$8
  Bottom 0.305: U5.37 64.77,29.21 64.77,31.75 58.42,38.1 44.83,38.1 37.85,45.09 P1.11 34.04,46.35
N$9
  Top 0.305: R7.2 PWR.+
N$10
  Top 0.305: RESET.+ R8.2
N$11
  Top 0.305: R30.1 46.23,23.62 Q2.1
N$12
  Top 0.305: J6.3 48.72,16.56 R24.1
N$13
  Top 0.305: J6.5 47.87,14.36 R25.1
N$14
  Top 0.305: R29.2 SD.+
N$18
  Top 0.305: R13.1 62.36,36.7 Q1.1
N$24  (via drill 0.3 pad 0.64)
  Top 0.305: U1.81 43,21.27 v42.55,21.72
  Bottom 0.305: P5.11 43.18,21.08 v42.55,21.72
N$32
  Top 0.305: U1.54 31.7,15.57 C19.2 C8.2
N$37
  Top 0.305: U1.71 40.2,15.3 R9.2 41.51,13.99 X2.3
RESET  (via drill 0.3 pad 0.64)
  Top 0.305: U1.38 26.29,24.77 C13.2 R2.2 v23.75,23.11 | RESET.- 14.48,5.08 20.32,5.08 | 20.32,5.08 20.45,5.08 RST.2 | 20.32,5.08 v20.32,5.71
  Bottom 0.305: v20.32,5.71 20.32,19.68 v23.75,23.11
SCK  (via drill 0.3 pad 0.64)
  Top 0.305: 49.4,35.69 R14.2 v48.26,35.56
  Bottom 0.305: v48.26,35.56 43.81,35.56 37.47,41.91 29.84,41.91 27.94,43.81 27.94,46.1 28.19,46.35 P2.MM
SCKP
  Bottom 0.305: P2.00 U5.14
SD  (via drill 0.3 pad 0.64)
  Top 0.305: SD.- 5.21,50.8 8.89,50.8 12.06,47.62 33.4,47.62 U5.11 37.85,52.07 43.18,52.07 43.81,51.44 43.81,40.01 v45.09,38.73 | v59.69,38.1 59.69,37.59 Q1.2
  Bottom 0.305: v45.09,38.73 59.05,38.73 v59.69,38.1
SD_CS
  Top 0.305: R12.1 49.14,17.66 J6.2 51.31,17.66 55.56,21.91 55.56,31.69 58.17,34.29 U8.4 61.47,34.29 61.59,34.42 Q1.3 61.59,34.67
SD_MISO  (via drill 0.3 pad 0.64)
  Top 0.305: R26.2 v45.09,12.95 | U8.5 58.12,34.94 56.83,33.66 v55.88,33.66
  Bottom 0.305: v55.88,33.66 55.88,13.97 54.86,12.95 v45.09,12.95
SPI_MOSI  (via drill 0.3 pad 0.64)
  Top 0.305: v45.09,17.53 R24.2 | U1.91 45.12,26.27 v45.28,26.42 | U8.3 58.22,33.64 56.2,31.62 56.2,21.78 v51.44,17.02
  Bottom 0.305: v51.44,17.02 45.59,17.02 v45.09,17.53 45.09,26.23 v45.28,26.42
SPI_SCK  (via drill 0.3 pad 0.64)
  Top 0.305: U1.90 45.7,25.77 v45.97,26.04 | v45.09,14.48 R25.2 | U8.8 53.88,36.29 v54.61,35.56
  Bottom 0.305: 55.24,23.11 55.24,34.92 v54.61,35.56 | 55.24,22.86 55.24,22.61 | 55.24,22.61 55.24,15.24 54.48,14.48 v45.09,14.48 | v45.97,26.04 45.97,23.88 46.99,22.86 54.99,22.86 | 54.99,22.86 55.24,22.86 | 54.99,22.86 55.24,23.11 | 54.99,22.86 55.24,22.61 | 55.24,22.86 55.24,23.11
V_OUT
  Top 0.305: U1.55 R4.2 30.67,11.68 V_OUT.1

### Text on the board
tPlace: Seeed
bPlace: Camera Shield | v1.0 07/28/2014 | by Seeed Studio | www.seeedstudio.com
bNames: D8 | CMR SPI_CS | HSUART | CMR_RX_TX | UART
